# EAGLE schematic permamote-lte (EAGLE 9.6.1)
AUTHOR: NEAL JACKSON; REV: C; TITLE: PERMAMOTE

## Sheet 1 of 5: NRF
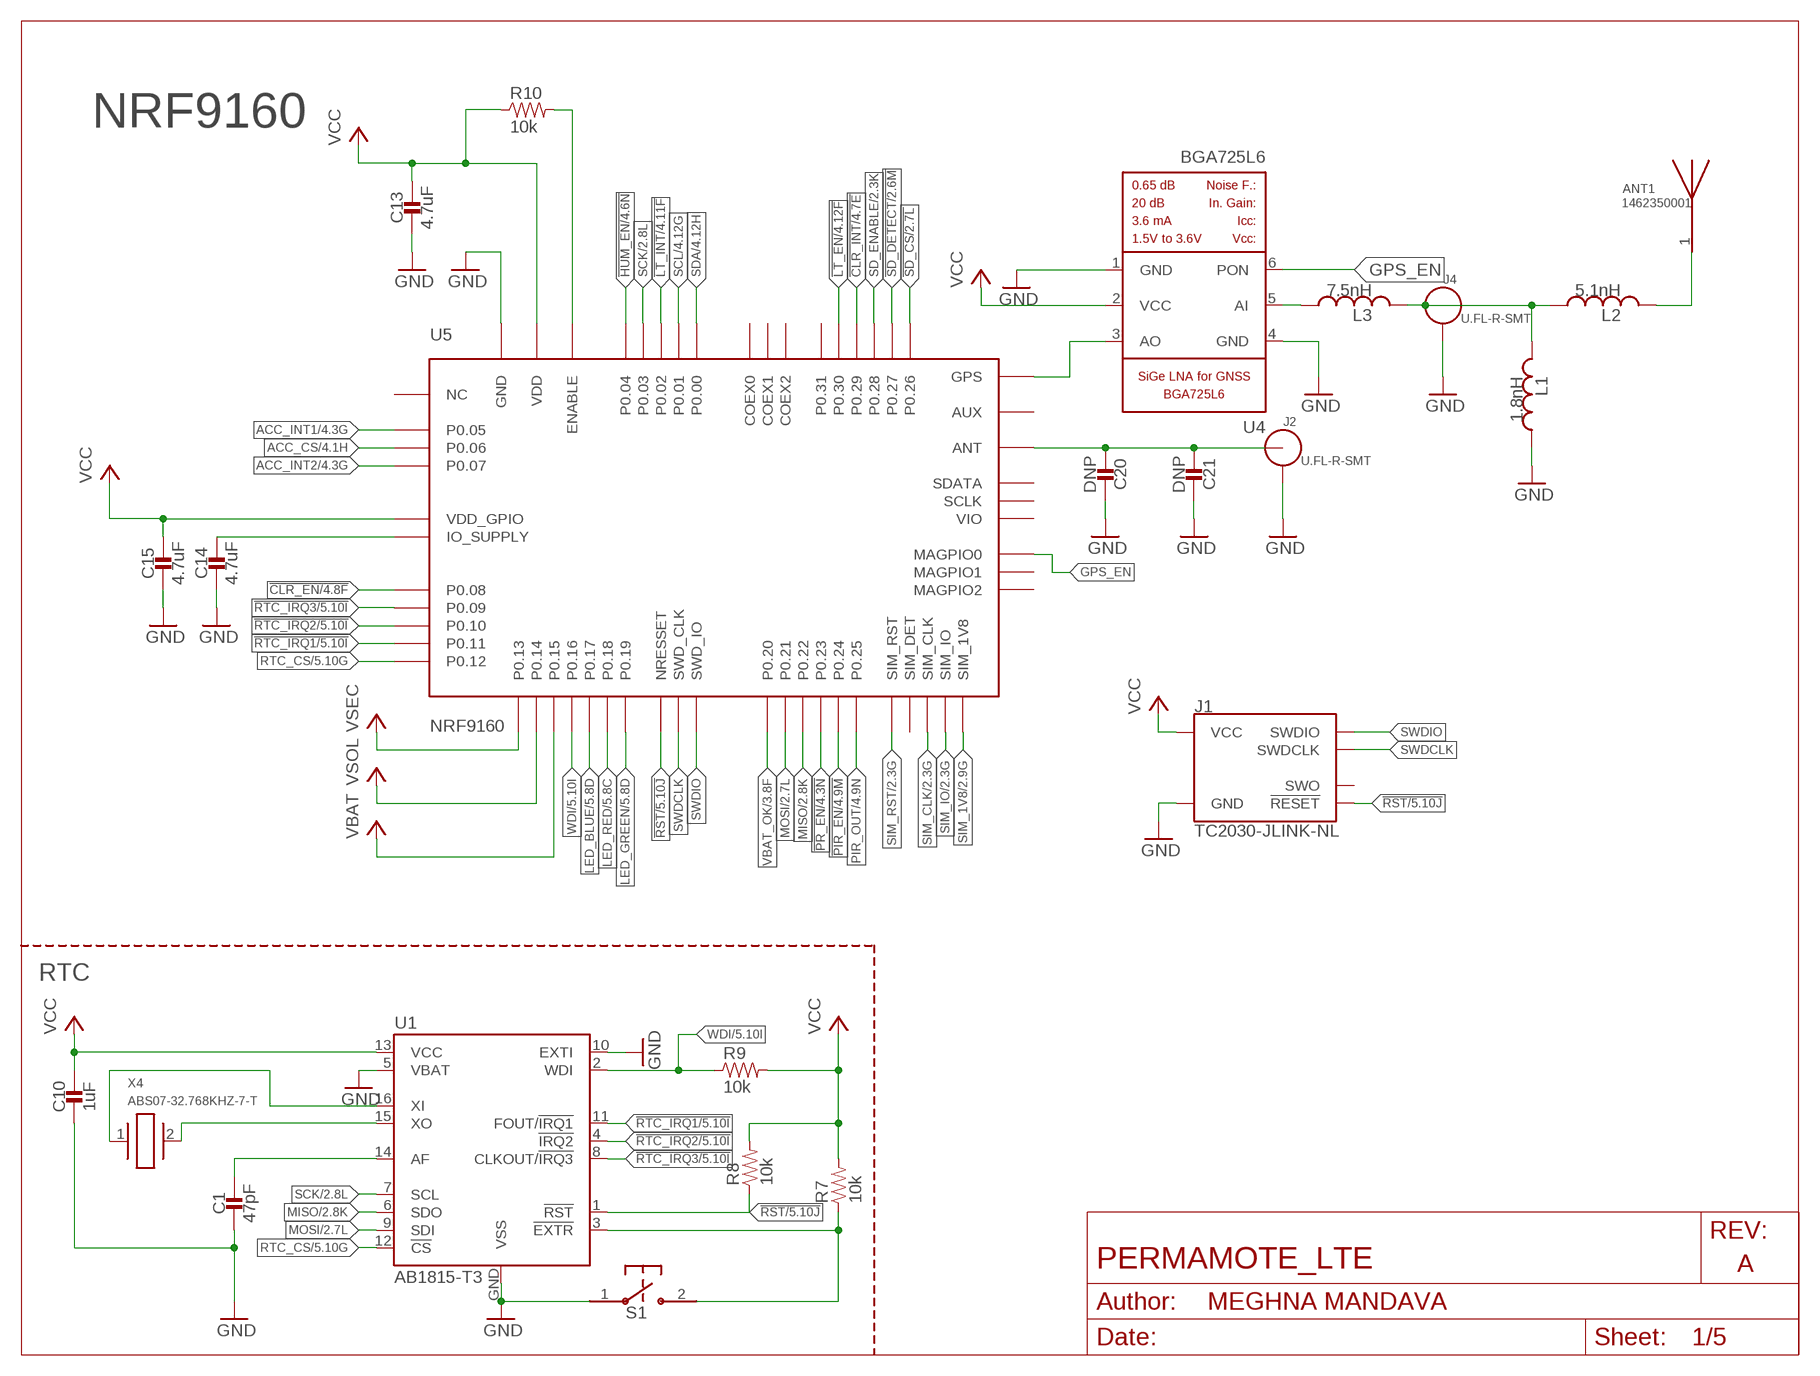
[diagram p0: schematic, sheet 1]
FRAME1 (LETTER_L_BLANK): AUTHOR: MEGHNA MANDAVA; REV: A; TITLE: PERMAMOTE_LTE

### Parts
ANT1  1462350001  [ANT_1462350001]
C1  47pF  CAPACITOR0402_CAP  [0402_CAP]
C10  1uF  CAPACITOR0402_CAP  [0402_CAP]
C13  4.7uF  CAPACITOR0402_CAP  [0402_CAP]
C14  4.7uF  CAPACITOR0402_CAP  [0402_CAP]
C15  4.7uF  CAPACITOR0402_CAP  [0402_CAP]
C20  DNP  CAPACITOR0402_CAP  [0402_CAP]
C21  DNP  CAPACITOR0402_CAP  [0402_CAP]
J1  TC2030-JLINK-NL  [TC2030-IDC-NL]
J2  U.FL-R-SMT  [U.FL_SMT]
J4  U.FL-R-SMT  [U.FL_SMT]
L1  1.8nH  INDUCTOR0402  [0402_CAP]
L2  5.1nH  INDUCTOR0402  [0402_CAP]
L3  7.5nH  INDUCTOR0402  [0402_CAP]
R7  10k  RESISTOR0402_RES  [0402_RES]
R8  10k  RESISTOR0402_RES  [0402_RES]
R9  10k  RESISTOR0402_RES  [0402_RES]
R10  10k  RESISTOR0402_RES  [0402_RES]
S1  B3U-1000P  [B3U-1000P]
U1  AB1815-T3  [QFN-16-3MM]
U4  BGA725L6  [LNA-TSLP-6-2-ORIG]
U5  NRF9160  [NRF9160]
X4  ABS07-32.768KHZ-7-T  [2-SMD]

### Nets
!CLR_EN: U5.P0.08 ; also sheet 4,5
!CLR_INT: U5.P0.29 ; also sheet 4,5
!HUM_EN: U5.P0.04 ; also sheet 4,5
!LT_EN: U5.P0.30 ; also sheet 4,5
!LT_INT: U5.P0.02 ; also sheet 4,5
!PIR_EN: U5.P0.24 ; also sheet 4,5
!PR_EN: U5.P0.23 ; also sheet 4,5
!RST: J1.3(!RESET) R8.1 U1.1(!RST) U5.NRESET(NRESSET) ; also sheet 5
!RTC_EXTR: R7.1 S1.2 U1.3(!EXTR)
!RTC_IRQ1: U1.11(FOUT/!IRQ1) U5.P0.11 ; also sheet 5
!RTC_IRQ2: U1.4(!IRQ2) U5.P0.10 ; also sheet 5
!RTC_IRQ3: U1.8(CLKOUT/!IRQ3) U5.P0.09 ; also sheet 5
!SD_CS: U5.P0.26 ; also sheet 2
!SD_DETECT: U5.P0.27 ; also sheet 2
ACC_CS: U5.P0.06 ; also sheet 4,5
ACC_INT1: U5.P0.05 ; also sheet 4,5
ACC_INT2: U5.P0.07 ; also sheet 4,5
GND: C1.2 C10.2 C13.2 C14.2 C15.2 C20.1 C21.1 J1.5(GND) J2.GND1 J2.GND2 J4.GND1 J4.GND2 L1.1 S1.1 U1.5(VBAT) U1.10(EXTI) U1.GND(VSS) U4.1(GND) U4.4(GND) U5.GND@1(GND) U5.GND@2(GND) U5.GND@3(GND) U5.GND@4(GND) U5.GND@5(GND) U5.GND@6(GND) U5.GND@7(GND) U5.GND@8(GND) U5.GND@9(GND) U5.GND@10(GND) U5.GND@11(GND) U5.GND@12(GND) U5.GND@13(GND) U5.GND@14(GND) U5.GND@15(GND) U5.GND@16(GND) U5.GND@17(GND) U5.GND@18(GND) U5.GND@19(GND) U5.GND@20(GND) U5.GND@21(GND) U5.GND@22(GND) U5.GND@23(GND) U5.GND@24(GND) U5.GND@25(GND) U5.GND@26(GND) U5.GND@27(GND) U5.GND@28(GND) U5.GND@29(GND) U5.GND@30(GND) U5.GND@31(GND) U5.GND@32(GND) U5.GND@33(GND) U5.GND@34(GND) U5.GND@35(GND) U5.GND_SHIELD@1(GND) U5.GND_SHIELD@2(GND) U5.GND_SHIELD@3(GND) U5.GND_SHIELD@4(GND) U5.GND_SHIELD@5(GND) U5.GND_SHIELD@6(GND) U5.GND_SHIELD@7(GND) U5.GND_SHIELD@8(GND) U5.GND_SHIELD@9(GND) U5.GND_SHIELD@10(GND) U5.GND_SHIELD@11(GND) U5.GND_SHIELD@12(GND) U5.GND_SHIELD@13(GND) U5.GND_SHIELD@14(GND) U5.GND_SHIELD@15(GND) U5.GND_SHIELD@16(GND) U5.GND_SHIELD@17(GND) U5.GND_SHIELD@18(GND) U5.GND_SHIELD@19(GND) U5.GND_SHIELD@20(GND) U5.GND_SHIELD@21(GND) U5.GND_SHIELD@22(GND) U5.GND_SHIELD@23(GND) U5.GND_SHIELD@24(GND) U5.GND_SHIELD@25(GND) U5.GND_SHIELD@26(GND) U5.GND_SHIELD@27(GND) U5.GND_SHIELD@28(GND) U5.GND_SHIELD@29(GND) U5.GND_SHIELD@30(GND) U5.GND_SHIELD@31(GND) U5.GND_SHIELD@32(GND) U5.GND_SHIELD@33(GND) U5.GND_SHIELD@34(GND) ; also sheet 2,3,4,5
GPS_EN: U4.6(PON) U5.MAGPIO0
LED_BLUE: U5.P0.17 ; also sheet 5
LED_GREEN: U5.P0.19 ; also sheet 5
LED_RED: U5.P0.18 ; also sheet 5
MISO: U1.6(SDO) U5.P0.22 ; also sheet 2,4,5
MOSI: U1.9(SDI) U5.P0.21 ; also sheet 2,4,5
N$1: U4.3(AO) U5.GPS
N$2: L3.1 U4.5(AI)
N$4: J4.SIG(ANT) L1.2 L2.1 L3.2
N$5: ANT1.1 L2.2
N$8: C20.2 C21.2 J2.SIG(ANT) U5.ANT
N$25: C1.1 U1.14(AF)
N$28: R10.2 U5.ENABLE
N$29: C14.1 U5.IO_SUPPLY
N$40: U1.15(XO) X4.2
N$43: U1.16(XI) X4.1
PIR_OUT: U5.P0.25 ; also sheet 4,5
RTC_CS: U1.12(!CS) U5.P0.12 ; also sheet 5
SCK: U1.7(SCL) U5.P0.03 ; also sheet 2,4,5
SCL: U5.P0.01 ; also sheet 4,5
SD_ENABLE: U5.P0.28 ; also sheet 2
SDA: U5.P0.00 ; also sheet 4,5
SIM_1V8: U5.SIM_1V8 ; also sheet 2
SIM_CLK: U5.SIM_CLK ; also sheet 2
SIM_IO: U5.SIM_IO ; also sheet 2
SIM_RST: U5.SIM_RST ; also sheet 2
SWDCLK: J1.4(SWDCLK) U5.SWDCLK(SWD_CLK)
SWDIO: J1.2(SWDIO) U5.SWDIO(SWD_IO)
VBAT: U5.P0.15 ; also sheet 3
VBAT_OK: U5.P0.20 ; also sheet 3
VCC: C10.1 C13.1 C15.1 J1.1(VCC) R7.2 R8.2 R9.2 R10.1 U1.13(VCC) U4.2(VCC) U5.VDD@1(VDD) U5.VDD@2(VDD) U5.VDD_GPIO ; also sheet 2,3,4,5
VSEC: U5.P0.13 ; also sheet 3
VSOL: U5.P0.14 ; also sheet 3,5
WDI: R9.1 U1.2(WDI) U5.P0.16 ; also sheet 5
Unconnected: J1.6(SWO) U5.AUX U5.COEX0 U5.COEX1 U5.COEX2 U5.MAGPIO1 U5.MAGPIO2 U5.NC1(NC) U5.NC2(NC) U5.NC3(NC) U5.NC4(NC) U5.NC5(NC) U5.NC6(NC) U5.NC7(NC) U5.NC8(NC) U5.NC9(NC) U5.NC10(NC) U5.NC11(NC) U5.NC12(NC) U5.NC13(NC) U5.NC14(NC) U5.NC15(NC) U5.NC16(NC) U5.NC17(NC) U5.NC18(NC) U5.NC19(NC) U5.NC20(NC) U5.NC21(NC) U5.NC22(NC) U5.NC23(NC) U5.NC24(NC) U5.NC25(NC) U5.NC26(NC) U5.NC27(NC) U5.NC28(NC) U5.NC29(NC) U5.NC30(NC) U5.NC31(NC) U5.NC32(NC) U5.NC33(NC) U5.NC34(NC) U5.NC35(NC) U5.P0.31 U5.SCLK U5.SDATA U5.SIM_DET U5.VIO

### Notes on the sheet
- NRF9160
- RTC

## Sheet 2 of 5: SIM and SD
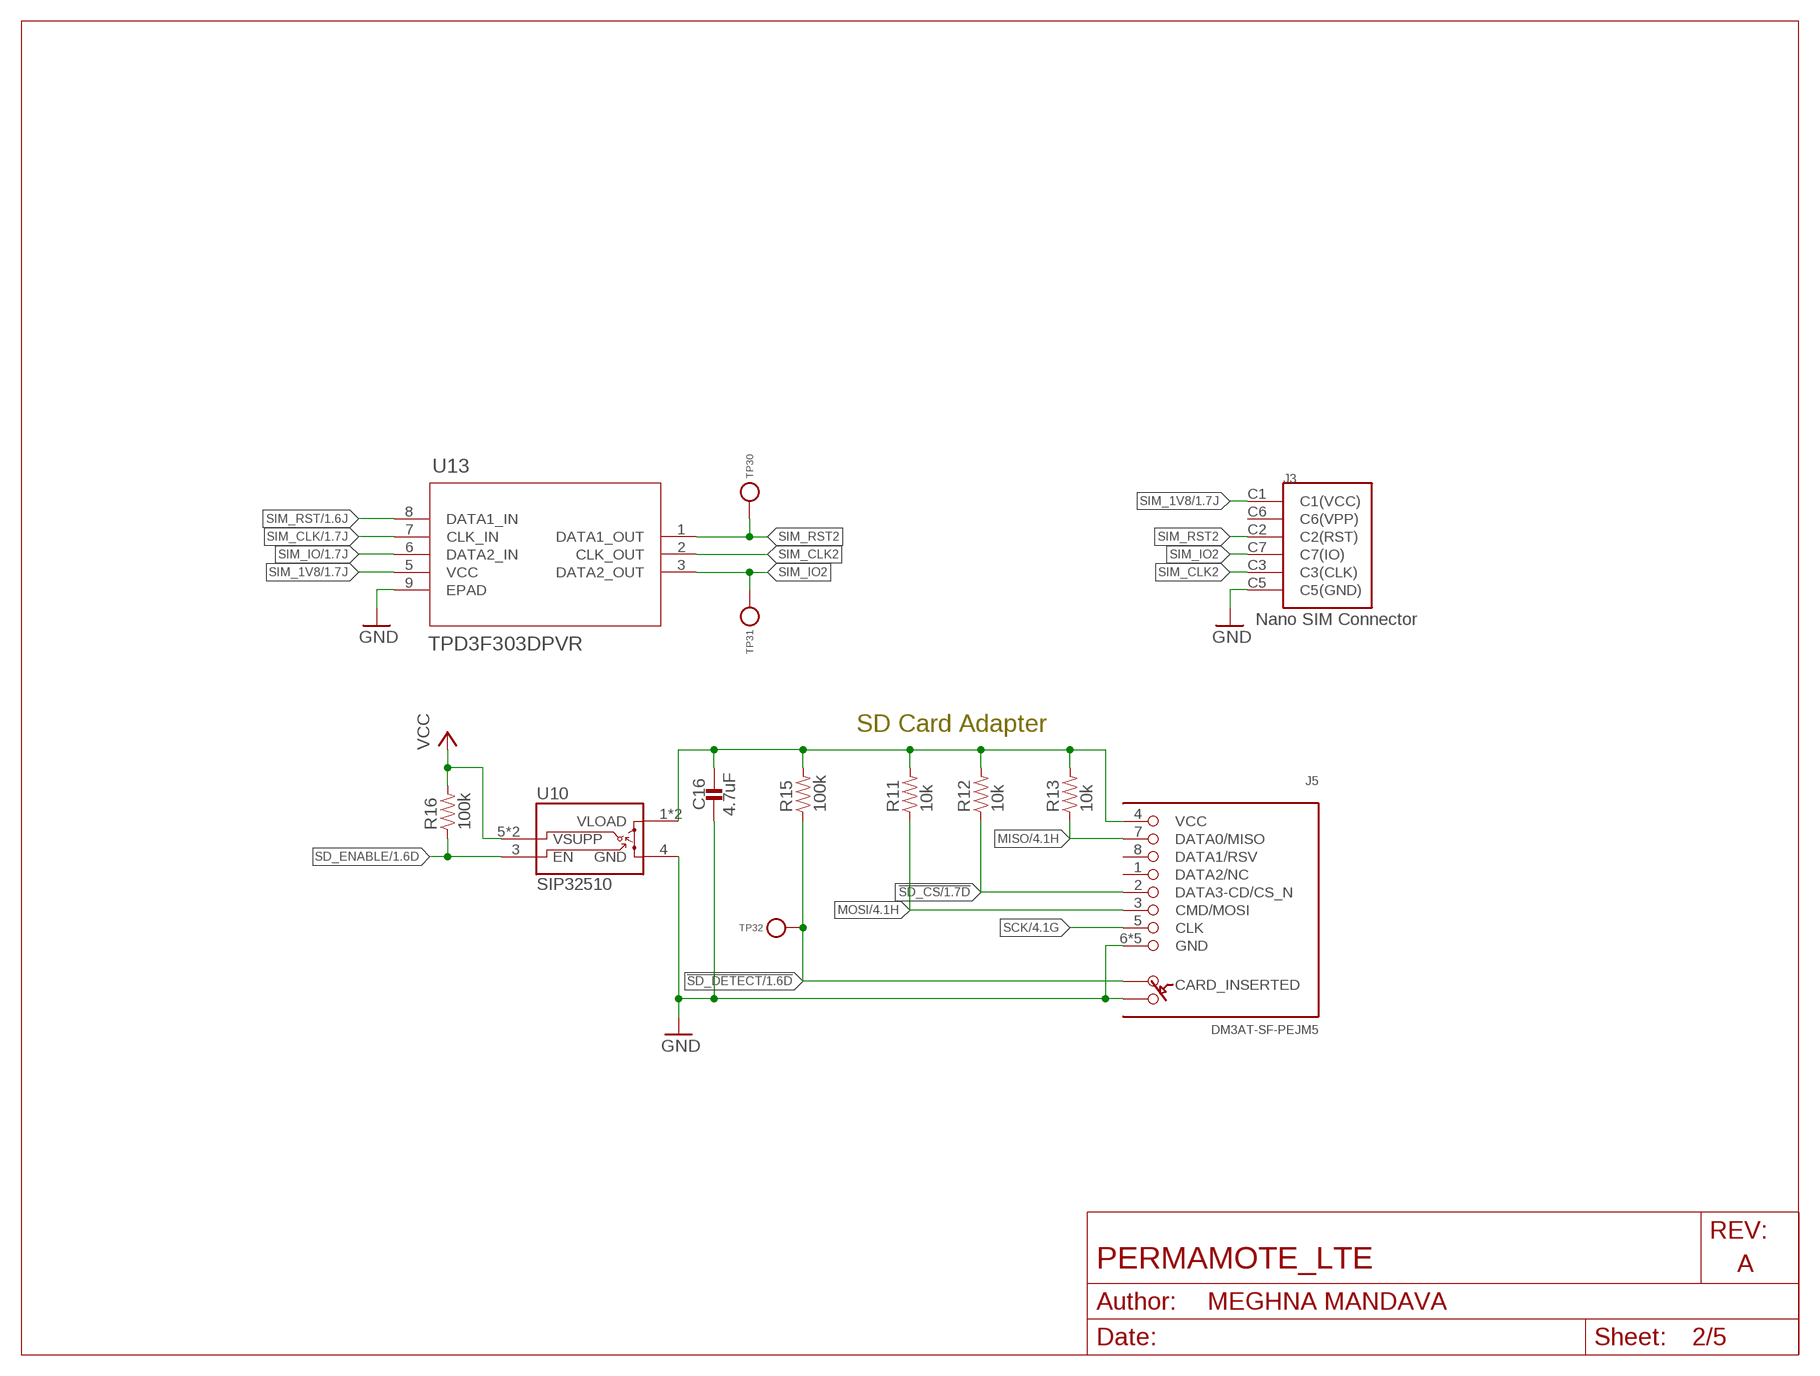
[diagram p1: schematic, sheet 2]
FRAME4 (LETTER_L_BLANK): AUTHOR: MEGHNA MANDAVA; REV: A; TITLE: PERMAMOTE_LTE

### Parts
C16  4.7uF  CAPACITOR0402_CAP  [0402_CAP]
J3  NANO_SIM  [WURTH_NANO_SIM]
J5  DM3AT-SF-PEJM5  [DM3AT-SF-PEJM5]
R11  10k  RESISTOR0402_RES  [0402_RES]
R12  10k  RESISTOR0402_RES  [0402_RES]
R13  10k  RESISTOR0402_RES  [0402_RES]
R15  100k  RESISTOR0402_RES  [0402_RES]
R16  100k  RESISTOR0402_RES  [0402_RES]
TP30  TEST-POINT  [PAD.03X.03]
TP31  TEST-POINT  [PAD.03X.03]
TP32  TEST-POINT  [PAD.03X.03]
U10  SIP32510  [TSOT23-6]
U13  TPD3F303DPVR  [DPV8_1P7X0P4]

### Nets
!SD_CS: J5.2(DATA3-CD/CS_N) R12.1 ; also sheet 1
!SD_DETECT: J5.A R15.1 TP32.P$1(TESTPOINT) ; also sheet 1
GND: C16.2 J3.C5(C5(GND)) J5.6(GND) J5.B J5.MOUNT0(GND) J5.MOUNT1(GND) J5.MOUNT2(GND) J5.MOUNT3(GND) U10.4(GND) U13.9(EPAD) ; also sheet 1,3,4,5
MISO: J5.7(DATA0/MISO) R13.1 ; also sheet 1,4,5
MOSI: J5.3(CMD/MOSI) R11.1 ; also sheet 1,4,5
N$13: C16.1 J5.4(VCC) R11.2 R12.2 R13.2 R15.2 U10.1(VLOAD) U10.2(VLOAD)
SCK: J5.5(CLK) ; also sheet 1,4,5
SD_ENABLE: R16.1 U10.3(EN) ; also sheet 1
SIM_1V8: J3.C1(C1(VCC)) U13.5(VCC) ; also sheet 1
SIM_CLK: U13.7(CLK_IN) ; also sheet 1
SIM_CLK2: J3.C3(C3(CLK)) U13.2(CLK_OUT)
SIM_IO: U13.6(DATA2_IN) ; also sheet 1
SIM_IO2: J3.C7(C7(IO)) TP31.P$1(TESTPOINT) U13.3(DATA2_OUT)
SIM_RST: U13.8(DATA1_IN) ; also sheet 1
SIM_RST2: J3.C2(C2(RST)) TP30.P$1(TESTPOINT) U13.1(DATA1_OUT)
VCC: R16.2 U10.5(VSUPP) U10.6(VSUPP) ; also sheet 1,3,4,5
Unconnected: J3.C6(C6(VPP)) J5.1(DATA2/NC) J5.8(DATA1/RSV)

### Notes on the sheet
- SD Card Adapter

## Sheet 3 of 5: Power supply
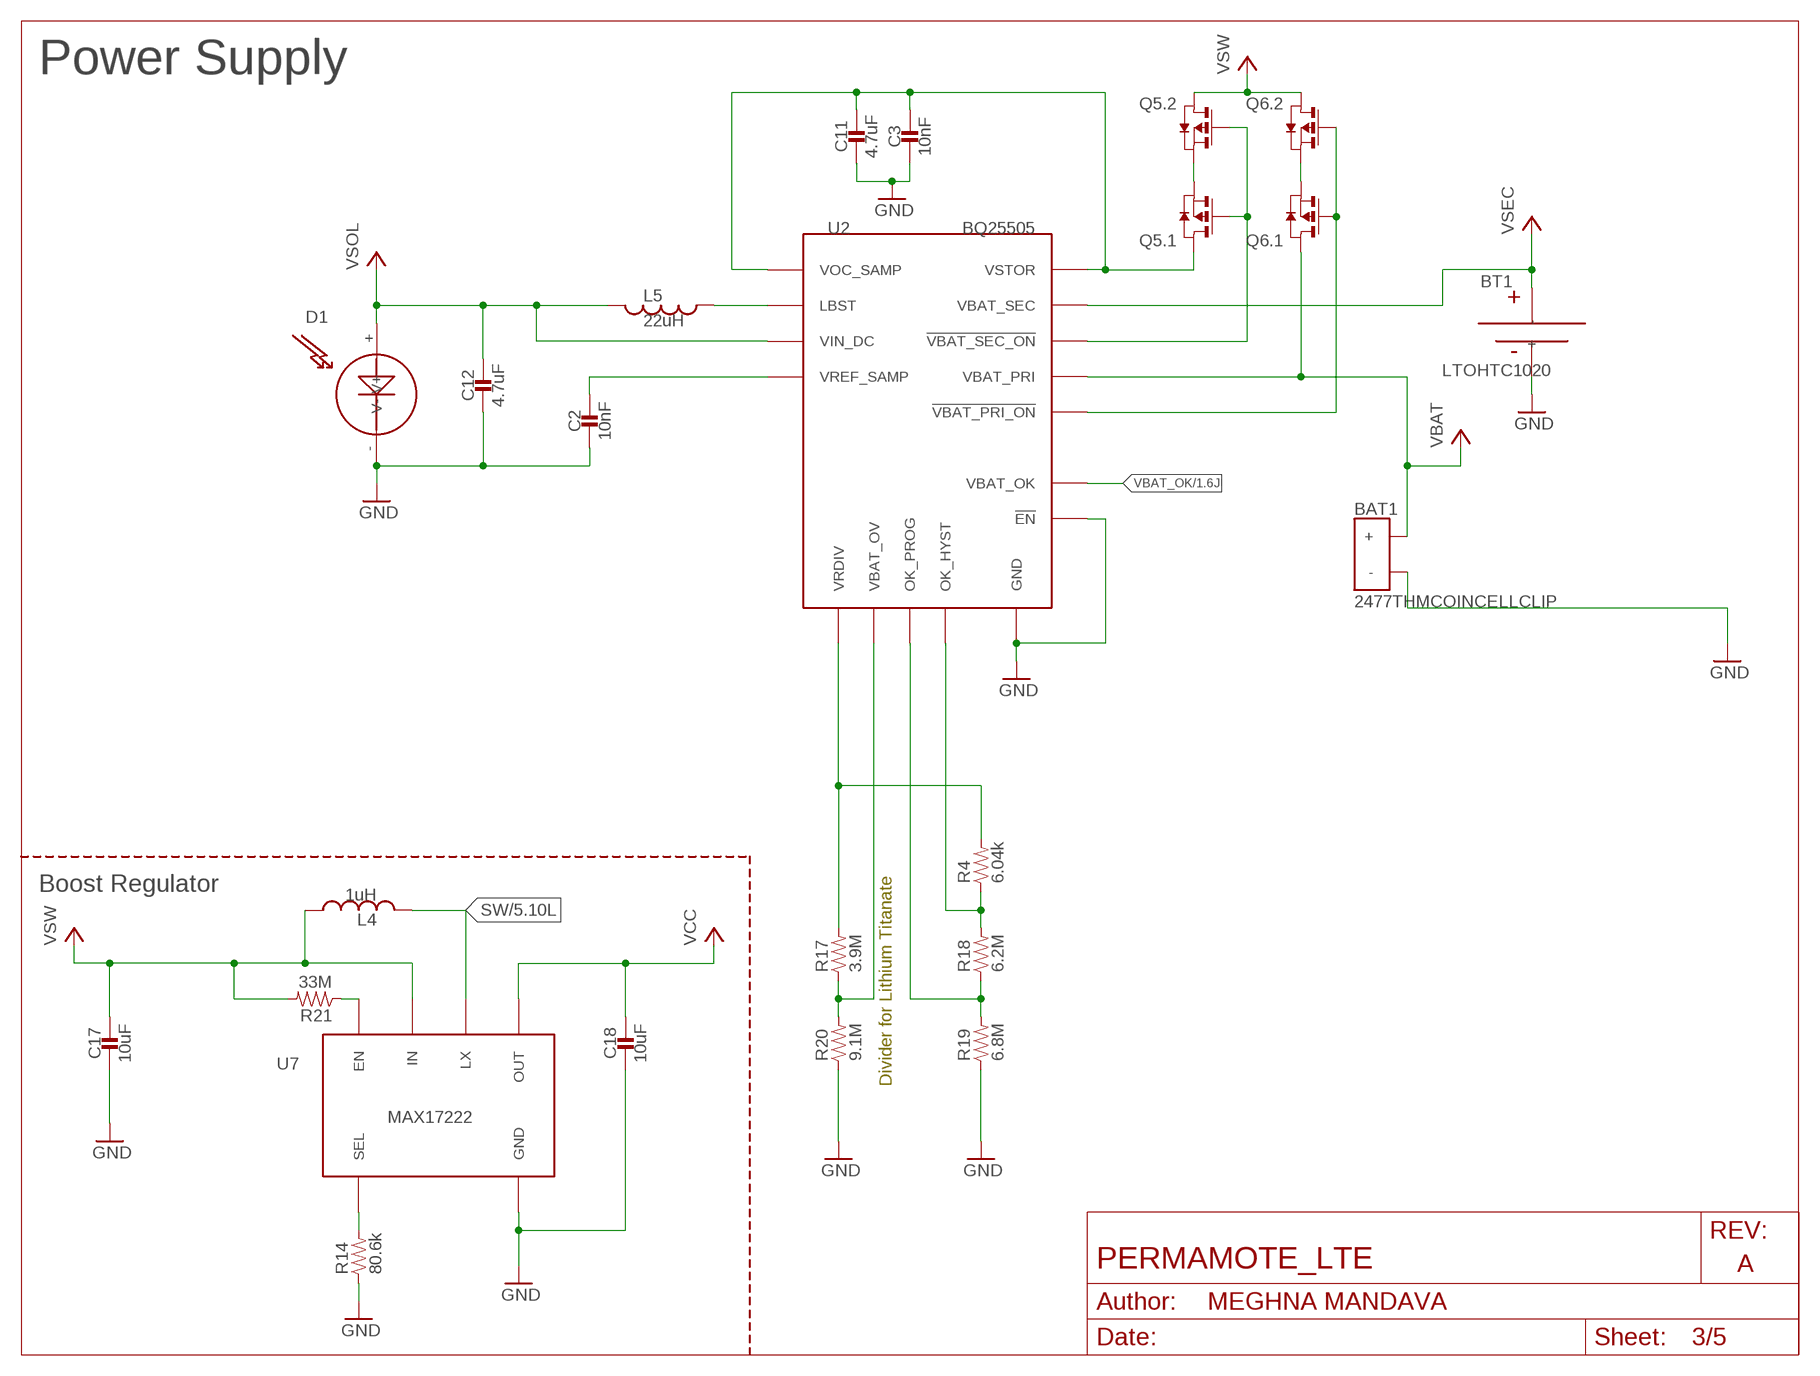
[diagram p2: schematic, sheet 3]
FRAME2 (LETTER_L_BLANK): AUTHOR: MEGHNA MANDAVA; REV: A; TITLE: PERMAMOTE_LTE

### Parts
BAT1  2477THMCOINCELLCLIP  [2477THMCOINCLIP]
BT1  LTOHTC1020  [1020]
C2  10nF  CAPACITOR0402_CAP  [0402_CAP]
C3  10nF  CAPACITOR0402_CAP  [0402_CAP]
C11  4.7uF  CAPACITOR0402_CAP  [0402_CAP]
C12  4.7uF  CAPACITOR0402_CAP  [0402_CAP]
C17  10uF  CAPACITOR0603_CAP  [0603_CAP]
C18  10uF  CAPACITOR0603_CAP  [0603_CAP]
D1  SOLARCELLHOLES  [SOLAR_HOLES]
L4  1uH  INDUCTORIHL  [IHL-1212BZ-11]
L5  22uH  INDUCTOR74437324220  [74437324220]
Q5  PMDXB950UPEL  [XDFN-6]
Q6  PMDXB950UPEL  [XDFN-6]
R4  6.04k  RESISTOR0402_RES  [0402_RES]
R14  80.6k  RESISTOR0603_RES  [0603-RES]
R17  3.9M  RESISTOR0402_RES  [0402_RES]
R18  6.2M  RESISTOR0402_RES  [0402_RES]
R19  6.8M  RESISTOR0402_RES  [0402_RES]
R20  9.1M  RESISTOR0402_RES  [0402_RES]
R21  33M  RESISTOR0603_RES  [0603-RES]
U2  BQ25505  [S-PVQFN-N20-RGR]
U7  MAX17222  [UDFN-6-MAXIM]

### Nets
!VBAT_PRI_ON: Q6.2(.1:G) Q6.5(.2:G) U2.10(!VBAT_PRI_ON)
!VBAT_SEC_ON: Q5.2(.1:G) Q5.5(.2:G) U2.9(!VBAT_SEC_ON)
GND: BAT1.GND(-) BT1.- C2.2 C3.2 C11.2 C12.2 C17.2 C18.2 D1.-(V-) R14.1 R19.1 R20.1 U2.1(GND) U2.5(!EN) U2.6(GND) U2.15(GND) U2.16(GND) U2.17(GND) U2.PAD(GND) U7.3(GND) ; also sheet 1,2,4,5
LBST: L5.P$1 U2.20(LBST)
N$12: R14.2 U7.4(SEL)
N$14: R21.1 U7.6(EN)
N$18: R17.1 R20.2 U2.7(VBAT_OV)
N$32: R4.2 R17.2 U2.8(VRDIV)
N$45: Q5.1(.1:S) Q5.4(.2:S)
N$53: Q6.1(.1:S) Q6.4(.2:S)
N$57: R18.1 R19.2 U2.12(OK_PROG)
N$58: R4.1 R18.2 U2.11(OK_HYST)
SW: L4.P$2 U7.2(LX) ; also sheet 5
VBAT: BAT1.1(+) BAT1.2(+) Q6.6(.1:D) U2.14(VBAT_PRI) ; also sheet 1
VBAT_OK: U2.13(VBAT_OK) ; also sheet 1
VCC: C18.1 U7.1(OUT) ; also sheet 1,2,4,5
VOC_SAMP_VSTOR: C3.1 C11.1 Q5.6(.1:D) U2.3(VOC_SAMP) U2.19(VSTOR)
VREF_SAMP: C2.1 U2.4(VREF_SAMP)
VSEC: BT1.+ U2.18(VBAT_SEC) ; also sheet 1
VSOL: C12.1 D1.+(V+) L5.P$2 U2.2(VIN_DC) ; also sheet 1,5
VSW: C17.1 L4.P$1 Q5.3(.2:D) Q6.3(.2:D) R21.2 U7.5(IN)

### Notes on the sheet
- Power Supply
- Boost Regulator
- Divider for Lithium Titanate

## Sheet 4 of 5: Sensors
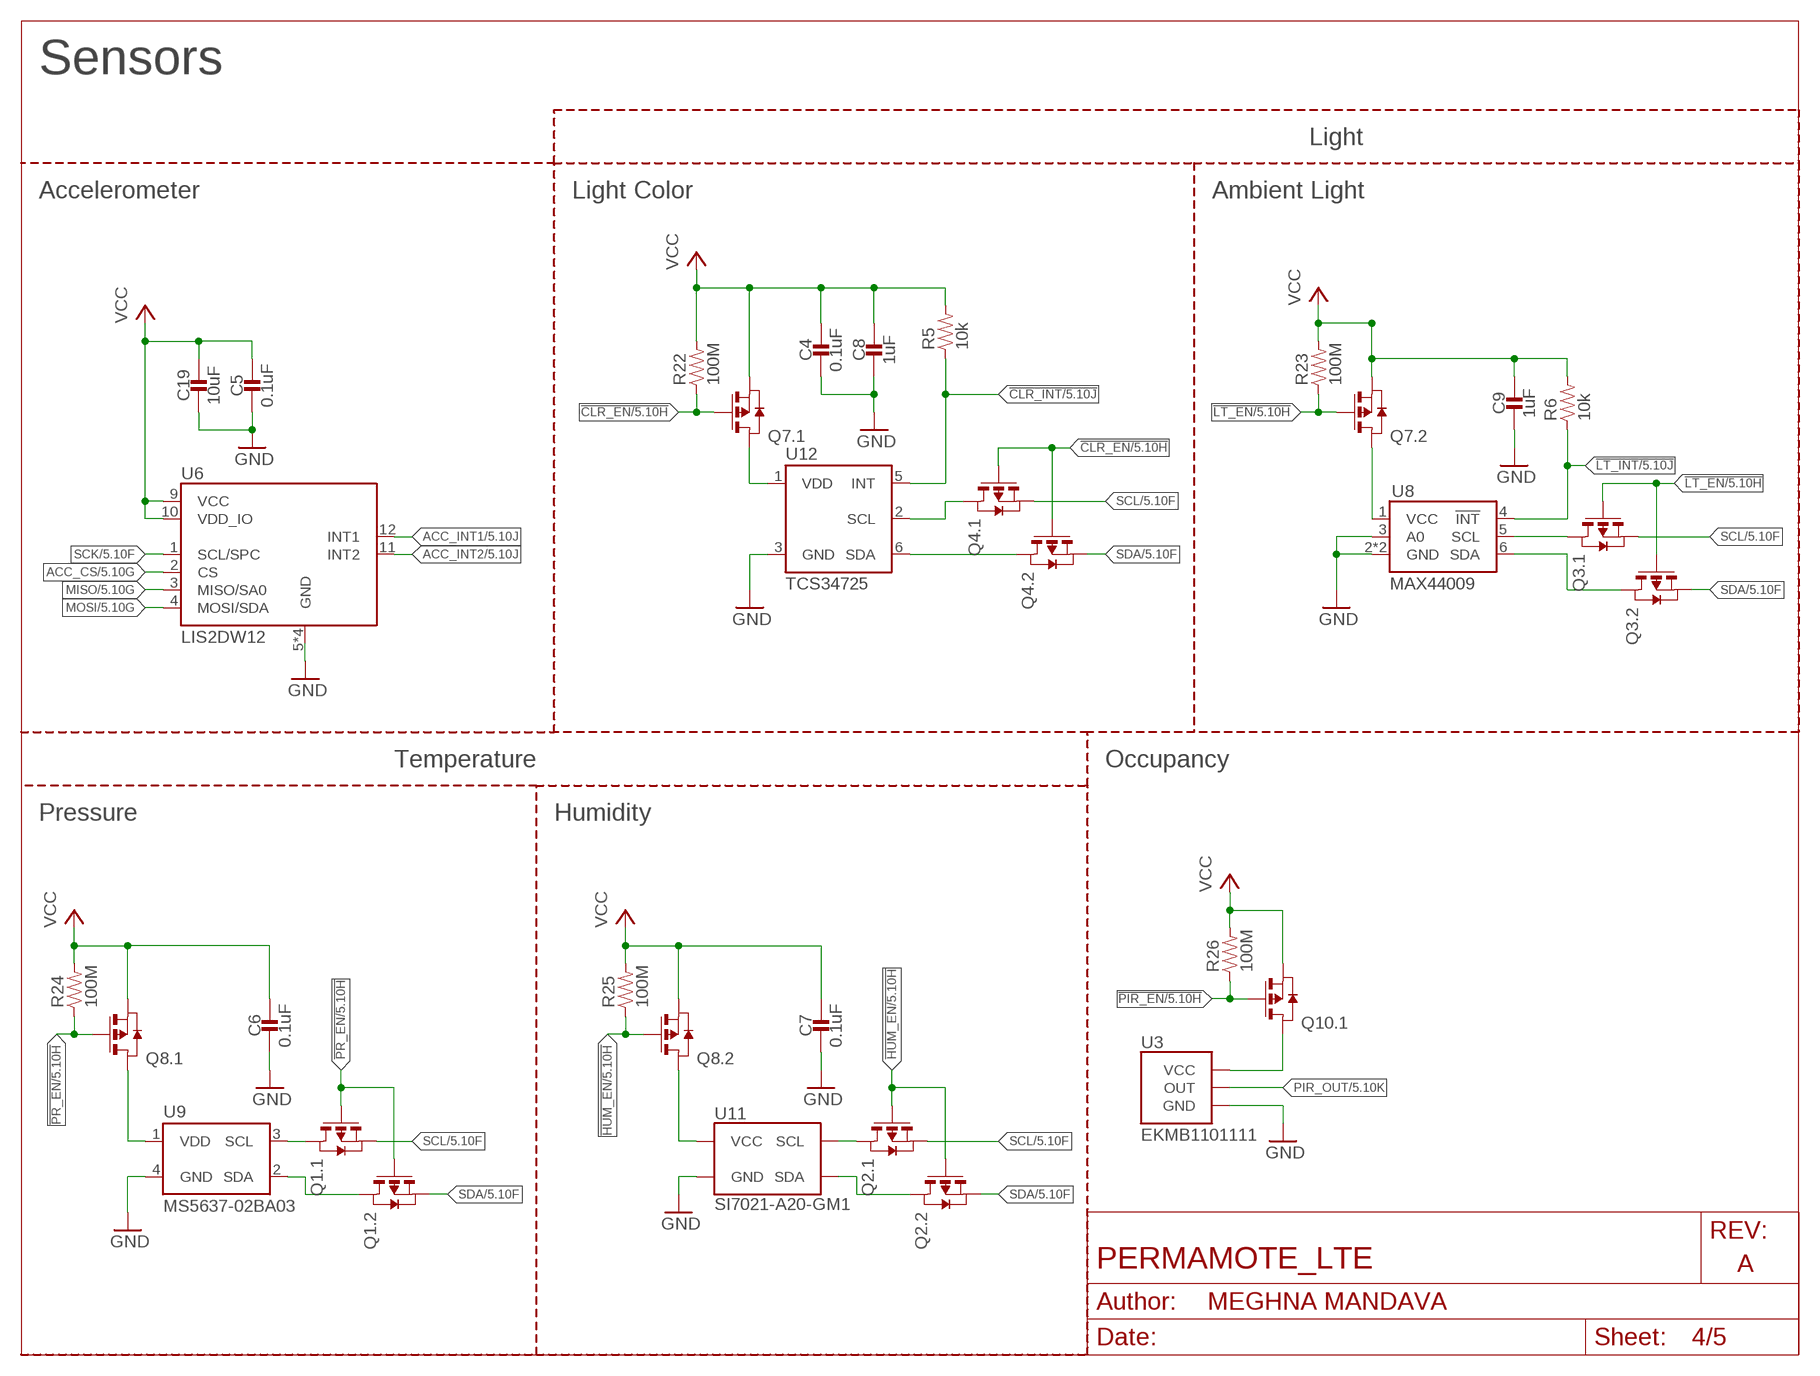
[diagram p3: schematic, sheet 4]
FRAME3 (LETTER_L_BLANK): AUTHOR: MEGHNA MANDAVA; REV: A; TITLE: PERMAMOTE_LTE

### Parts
C4  0.1uF  CAPACITOR0402_CAP  [0402_CAP]
C5  0.1uF  CAPACITOR0402_CAP  [0402_CAP]
C6  0.1uF  CAPACITOR0402_CAP  [0402_CAP]
C7  0.1uF  CAPACITOR0402_CAP  [0402_CAP]
C8  1uF  CAPACITOR0402_CAP  [0402_CAP]
C9  1uF  CAPACITOR0402_CAP  [0402_CAP]
C19  10uF  CAPACITOR0603_CAP  [0603_CAP]
Q1  PMDXB950UPEL  [XDFN-6]
Q2  PMDXB950UPEL  [XDFN-6]
Q3  PMDXB950UPEL  [XDFN-6]
Q4  PMDXB950UPEL  [XDFN-6]
Q7  PMDXB950UPEL  [XDFN-6]
Q8  PMDXB950UPEL  [XDFN-6]
Q10  PMDXB950UPEL  [XDFN-6]
R5  10k  RESISTOR0402_RES  [0402_RES]
R6  10k  RESISTOR0402_RES  [0402_RES]
R22  100M  RESISTOR0402_RES  [0402_RES]
R23  100M  RESISTOR0402_RES  [0402_RES]
R24  100M  RESISTOR0402_RES  [0402_RES]
R25  100M  RESISTOR0402_RES  [0402_RES]
R26  100M  RESISTOR0402_RES  [0402_RES]
U3  EKMB1101111  [AMN2]
U6  LIS2DW12  [LGA-12]
U8  MAX44009  [UDFN-6-EXPOSED]
U9  MS5637-02BA03  [4-SMD]
U11  SI7021-A20-GM1  [DFN-6/3MM]
U12  TCS34725  [FN-6]

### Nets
!CLR_EN: Q4.2(.1:G) Q4.5(.2:G) Q7.2(.1:G) R22.1 ; also sheet 1,5
!CLR_INT: R5.1 U12.5(INT) ; also sheet 1,5
!HUM_EN: Q2.2(.1:G) Q2.5(.2:G) Q8.5(.2:G) R25.1 ; also sheet 1,5
!LT_EN: Q3.2(.1:G) Q3.5(.2:G) Q7.5(.2:G) R23.1 ; also sheet 1,5
!LT_INT: R6.1 U8.4(!INT) ; also sheet 1,5
!PIR_EN: Q10.2(.1:G) R26.1 ; also sheet 1,5
!PR_EN: Q1.2(.1:G) Q1.5(.2:G) Q8.2(.1:G) R24.1 ; also sheet 1,5
ACC_CS: U6.2(CS) ; also sheet 1,5
ACC_INT1: U6.12(INT1) ; also sheet 1,5
ACC_INT2: U6.11(INT2) ; also sheet 1,5
GND: C4.2 C5.2 C6.2 C7.2 C8.2 C9.2 C19.2 U3.GND U6.5(GND) U6.6(GND) U6.7(GND) U6.8(GND) U8.2(GND) U8.3(A0) U8.EP(GND) U9.4(GND) U11.2(GND) U12.3(GND) ; also sheet 1,2,3,5
MISO: U6.3(MISO/SA0) ; also sheet 1,2,5
MOSI: U6.4(MOSI/SDA) ; also sheet 1,2,5
N$20: Q7.3(.2:D) U8.1(VCC)
N$21: Q8.6(.1:D) U9.1(VDD)
N$22: Q8.3(.2:D) U11.5(VCC)
N$23: Q10.6(.1:D) U3.VCC
N$31: Q7.6(.1:D) U12.1(VDD)
N$34: Q1.6(.1:D) U9.3(SCL)
N$41: Q1.3(.2:D) U9.2(SDA)
N$48: Q2.3(.2:D) U11.1(SDA)
N$50: Q2.6(.1:D) U11.6(SCL)
N$51: Q3.3(.2:D) U8.6(SDA)
N$52: Q3.6(.1:D) U8.5(SCL)
N$54: Q4.3(.2:D) U12.6(SDA)
N$55: Q4.6(.1:D) U12.2(SCL)
PIR_OUT: U3.OUT ; also sheet 1,5
SCK: U6.1(SCL/SPC) ; also sheet 1,2,5
SCL: Q1.1(.1:S) Q2.1(.1:S) Q3.1(.1:S) Q4.1(.1:S) ; also sheet 1,5
SDA: Q1.4(.2:S) Q2.4(.2:S) Q3.4(.2:S) Q4.4(.2:S) ; also sheet 1,5
VCC: C4.1 C5.1 C6.1 C7.1 C8.1 C9.1 C19.1 Q7.1(.1:S) Q7.4(.2:S) Q8.1(.1:S) Q8.4(.2:S) Q10.1(.1:S) R5.2 R6.2 R22.2 R23.2 R24.2 R25.2 R26.2 U6.9(VCC) U6.10(VDD_IO) ; also sheet 1,2,3,5
Unconnected: Q10.3(.2:D) Q10.4(.2:S) Q10.5(.2:G)

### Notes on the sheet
- Sensors
- Light
- Accelerometer | Light Color | Ambient Light
- Temperature | Occupancy
- Pressure | Humidity

## Sheet 5 of 5: Debugging
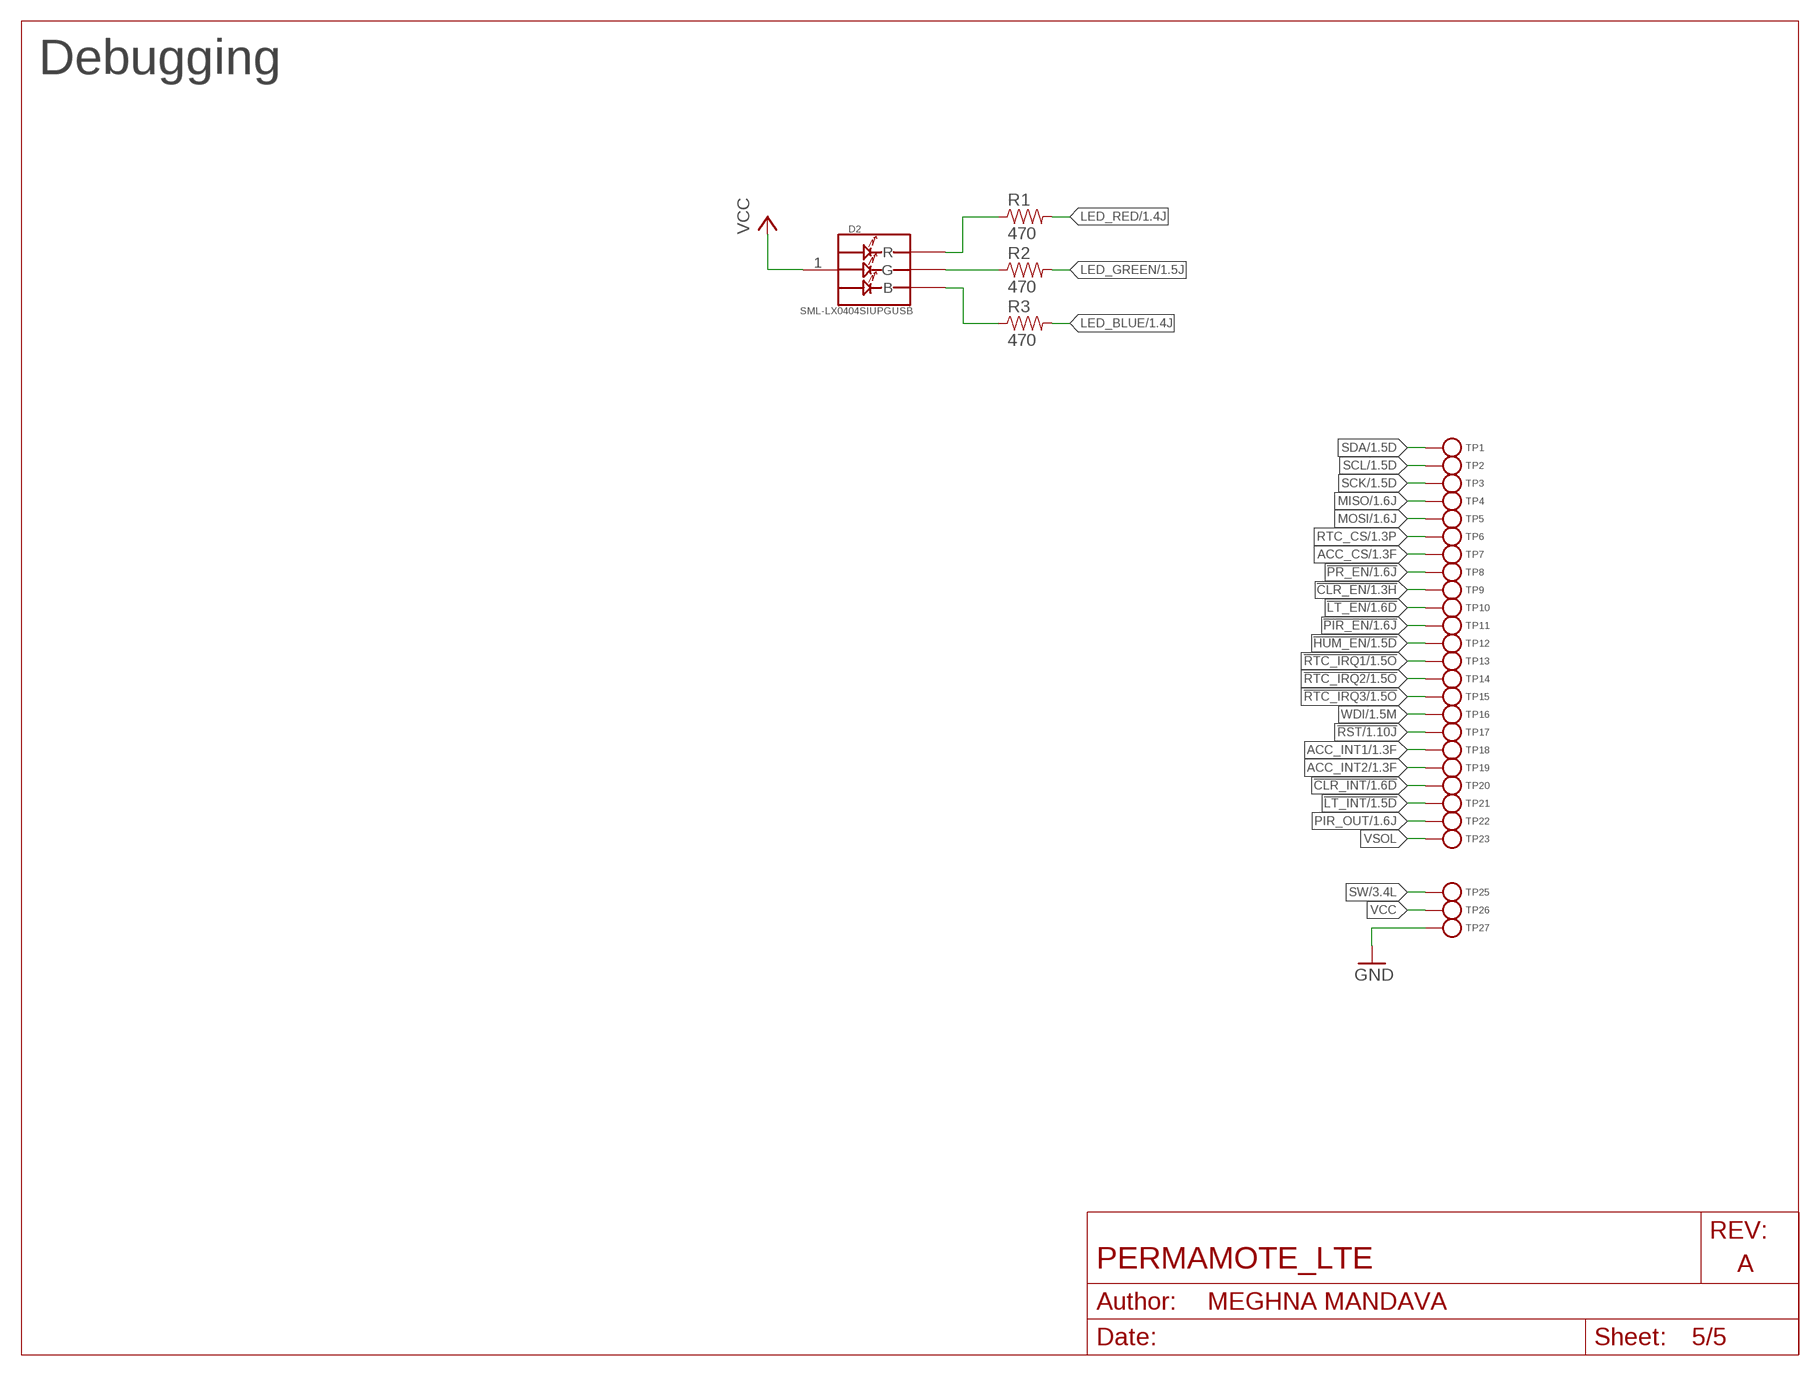
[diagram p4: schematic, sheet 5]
FRAME5 (LETTER_L_BLANK): AUTHOR: MEGHNA MANDAVA; REV: A; TITLE: PERMAMOTE_LTE

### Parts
D2  SML-LX0404SIUPGUSB  [1MM_SQ_4PAD]
R1  470  RESISTOR0402_RES  [0402_RES]
R2  470  RESISTOR0402_RES  [0402_RES]
R3  470  RESISTOR0402_RES  [0402_RES]
TP1  TEST-POINT  [PAD.03X.03]
TP2  TEST-POINT  [PAD.03X.03]
TP3  TEST-POINT  [PAD.03X.03]
TP4  TEST-POINT  [PAD.03X.03]
TP5  TEST-POINT  [PAD.03X.03]
TP6  TEST-POINT  [PAD.03X.03]
TP7  TEST-POINT  [PAD.03X.03]
TP8  TEST-POINT  [PAD.03X.03]
TP9  TEST-POINT  [PAD.03X.03]
TP10  TEST-POINT  [PAD.03X.03]
TP11  TEST-POINT  [PAD.03X.03]
TP12  TEST-POINT  [PAD.03X.03]
TP13  TEST-POINT  [PAD.03X.03]
TP14  TEST-POINT  [PAD.03X.03]
TP15  TEST-POINT  [PAD.03X.03]
TP16  TEST-POINT  [PAD.03X.03]
TP17  TEST-POINT  [PAD.03X.03]
TP18  TEST-POINT  [PAD.03X.03]
TP19  TEST-POINT  [PAD.03X.03]
TP20  TEST-POINT  [PAD.03X.03]
TP21  TEST-POINT  [PAD.03X.03]
TP22  TEST-POINT  [PAD.03X.03]
TP23  TEST-POINT  [PAD.03X.03]
TP25  TEST-POINT  [PAD.03X.03]
TP26  TEST-POINT  [PAD.03X.03]
TP27  TEST-POINT  [PAD.03X.03]

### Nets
!CLR_EN: TP9.P$1(TESTPOINT) ; also sheet 1,4
!CLR_INT: TP20.P$1(TESTPOINT) ; also sheet 1,4
!HUM_EN: TP12.P$1(TESTPOINT) ; also sheet 1,4
!LT_EN: TP10.P$1(TESTPOINT) ; also sheet 1,4
!LT_INT: TP21.P$1(TESTPOINT) ; also sheet 1,4
!PIR_EN: TP11.P$1(TESTPOINT) ; also sheet 1,4
!PR_EN: TP8.P$1(TESTPOINT) ; also sheet 1,4
!RST: TP17.P$1(TESTPOINT) ; also sheet 1
!RTC_IRQ1: TP13.P$1(TESTPOINT) ; also sheet 1
!RTC_IRQ2: TP14.P$1(TESTPOINT) ; also sheet 1
!RTC_IRQ3: TP15.P$1(TESTPOINT) ; also sheet 1
ACC_CS: TP7.P$1(TESTPOINT) ; also sheet 1,4
ACC_INT1: TP18.P$1(TESTPOINT) ; also sheet 1,4
ACC_INT2: TP19.P$1(TESTPOINT) ; also sheet 1,4
GND: TP27.P$1(TESTPOINT) ; also sheet 1,2,3,4
LED_BLUE: R3.2 ; also sheet 1
LED_GREEN: R2.2 ; also sheet 1
LED_RED: R1.2 ; also sheet 1
MISO: TP4.P$1(TESTPOINT) ; also sheet 1,2,4
MOSI: TP5.P$1(TESTPOINT) ; also sheet 1,2,4
N$15: D2.2(R) R1.1
N$17: D2.4(G) R2.1
N$19: D2.3(B) R3.1
PIR_OUT: TP22.P$1(TESTPOINT) ; also sheet 1,4
RTC_CS: TP6.P$1(TESTPOINT) ; also sheet 1
SCK: TP3.P$1(TESTPOINT) ; also sheet 1,2,4
SCL: TP2.P$1(TESTPOINT) ; also sheet 1,4
SDA: TP1.P$1(TESTPOINT) ; also sheet 1,4
SW: TP25.P$1(TESTPOINT) ; also sheet 3
VCC: D2.1(VDD) TP26.P$1(TESTPOINT) ; also sheet 1,2,3,4
VSOL: TP23.P$1(TESTPOINT) ; also sheet 1,3
WDI: TP16.P$1(TESTPOINT) ; also sheet 1

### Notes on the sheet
- Debugging

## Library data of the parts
ANT1 = chips:1462350001: Antenna GPS 1.4dBi Gain 1578MHz SMD T/R; DESCRIPTION: Antenna GPS 1.4dBi Gain 1578MHz SMD T/R; DIGI-KEY_PART_NUMBER: WM15009CT-ND; DIGI-KEY_PURCHASE_URL: https://www.digikey.com/product-detail/en/molex/1462350001/WM15009CT-ND/6159255?utm_source=snapeda&utm_medium=aggregator&utm_campaign=symbol; DIGIKEY: WM15009CT-ND; MF: Molex; MP: 1462350001; MPN: 1462350001; PACKAGE: None
BAT1 = batteries:2477THMCOINCELLCLIP: Battery clip for 2477 Coin Cell; DIGIKEY: 36-3039-ND; MANUFACTURER: Keystone; MPN: 3039
BT1 = batteries:LTOHTC
C1 = passives:CAPACITOR: SMD Capacitor; DIGIKEY: 490-5942-1-ND; MPN: GRM1555C1H470JA01D
C2 C3 = passives:CAPACITOR: SMD Capacitor; DIGIKEY: 490-4516-1-ND; MPN: GRM155R71H103KA88D
C4-C7 = passives:CAPACITOR: SMD Capacitor; DIGIKEY: 490-6328-1-ND; MPN: GRM155R71C104KA88J
C8-C10 = passives:CAPACITOR: SMD Capacitor; DIGIKEY: 490-7195-1-ND; MPN: GRM155R70G105KA12D
C11-C15 = passives:CAPACITOR: SMD Capacitor; DIGIKEY: 445-5947-1-ND; MPN: C1005X5R0J475K050BC
C16 = passives:CAPACITOR: SMD Capacitor; DESCRIPTION: CAP CER 4.7UF 10V X5R 0402; DIGIKEY: 1276-1480-1-ND; MANUFACTURER: Samsung Electro-Mechanics; MPN: CL05A475KP5NRNC
C17-C19 = passives:CAPACITOR: SMD Capacitor; DIGIKEY: 490-3896-1-ND; MPN: GRM188R60J106ME47D
C20 C21 = passives:CAPACITOR: SMD Capacitor
D1 = permamote:SOLARCELL: Generic solar cell; DIGIKEY: 869-1001-ND; MPN: AM-1454CA
D2 = leds:SML-LX0404SIUPGUSB: 1mm^2 RGB LED; DIGIKEY: 67-2125-1-ND; MANUFACTURER: Lumex Opto; MPN: SML-LX0404SIUPGUSB
J1 = connector:TC2030-JLINK
J2 J4 = connector:U.FL-R-SMT: U.FL-R-SMT Antenna Connector; DIGIKEY: H122041-ND; MANUFACTURER: Hirose; MPN: U.FL-R-SMT-1(01)
J3 = signpost:NANO_SIM: WURTH Nano SIM Connector; DIGIKEY: 732-5954-1-ND; MANUFACTURER: Wurth; MPN: 693043020611
J5 = connector:DM3AT-SF-PEJM5: CONN MICRO SD R/A PUSH-PUSH SMD; DESCRIPTION: CONN MICRO SD CARD PUSH-PUSH R/A; DIGIKEY: HR1964CT-ND; MANUFACTURER: Hirose Electric Co Ltd; MPN: DM3AT-SF-PEJM5
L1 = passives:INDUCTOR: A very specific inductor; DIGIKEY: 490-2613-1-ND; MPN: LQG15HS1N8S02D
L2 = passives:INDUCTOR: A very specific inductor; DIGIKEY: 490-6564-1-ND; MPN: LQG15HN5N1S02D
L3 = passives:INDUCTOR: A very specific inductor; DIGIKEY: 490-6565-1-ND; MPN: LQG15HN7N5J02D
L4 = passives:INDUCTOR: A very specific inductor; DIGIKEY: 541-1319-1-ND; MANUFACTURER: Vishay Dale; MPN: IHLP1212BZER1R0M11
L5 = passives:INDUCTOR: A very specific inductor; DIGIKEY: 732-3340-1-ND; MPN: 74437324220
Q1-Q8 Q10 = fets:PMDXB950UPEL: 20 V 500mA, dual P-channel Trench MOSFET; DIGIKEY: 1727-2601-1-ND; MANUFACTURER: NEXPERIA; MPN: PMDXB950UPELZ
R1-R3 = passives:RESISTOR: Resistor; DIGIKEY: 311-470JRCT-ND; MPN: RC0402JR-07470RL
R4 = passives:RESISTOR: Resistor; DIGIKEY: YAG2293CT-ND; MPN: RC0402FR-076K04L
R5-R10 = passives:RESISTOR: Resistor; DIGIKEY: 311-10KJRCT-ND; MPN: RC0402JR-0710KL
R11-R13 = passives:RESISTOR: Resistor; DESCRIPTION: RES SMD 10K OHM 1% 1/16W 0402; DIGIKEY: 1276-3431-1-ND; MANUFACTURER: Samsung Electro-Mechanics; MPN: RC1005F103CS
R14 = passives:RESISTOR: Resistor; DIGIKEY: 311-80.6KHRCT-ND; MPN: RC0603FR-0780K6L
R15 R16 = passives:RESISTOR: Resistor; DESCRIPTION: RES SMD 100K OHM 1% 1/5W 0402; DIGIKEY: 541-100KYCT-ND; MANUFACTURER: Vishay Dale; MPN: CRCW0402100KFKEDHP
R17 = passives:RESISTOR: Resistor; DIGIKEY: YAG3301CT-ND; MPN: RC0402JR-073M9L
R18 = passives:RESISTOR: Resistor; DIGIKEY: YAG3309CT-ND; MPN: RC0402JR-076M2L
R19 = passives:RESISTOR: Resistor; DIGIKEY: YAG3310CT-ND; MPN: RC0402JR-076M8L
R20 = passives:RESISTOR: Resistor; DIGIKEY: YAG3322CT-ND; MPN: RC0402JR-079M1L
R21 = passives:RESISTOR: Resistor; DIGIKEY: HMC0603JT33M0CT-ND; MPN: HMC0603JT33M0
R22-R26 = passives:RESISTOR: Resistor; DIGIKEY: 541-100MAHCT-ND; MPN: HMC0402JT100M
S1 = switches:B3U: Switch; DIGIKEY: SW1020CT-ND; MANUFACTURER: Omron; MPN: B3U-1000P
TP1-TP23 TP25-TP27 TP30-TP32 = headers:TEST-POINT
U1 = chips:AB1815-T3: Ultra-low current RTC. 55nA quiescent @ 3V. 1.5-3.6V input.; DIGIKEY: 535-11936-1-ND; MANUFACTURER: Abracon; MPN: AB1815-T3
U2 = chips:BQ25505: EH front end for switching between primary and secondary cells; DIGIKEY: 296-37078-1-ND; MANUFACTURER: TI; MPN: BQ25505RGRR
U3 = chips:EKMB: Passive infrared human detection sensor with built-in amp.; DIGIKEY: 255-3065-ND; MANUFACTURER: PANASONIC; MPN: EKMB1101111
U4 = chips:BGA725L6; DIGIKEY: BGA725L6E6327FTSA1CT-ND; MANUFACTURER: Infineon Technologies; MPN: BGA725L6E6327FTSA1
U5 = chips:NRF9160; DIGIKEY: 1490-1076-1-ND; MANUFACTURER: Nordic Semiconductor; MPN: NRF9160-SICA-R7
U6 = chips:LIS2DW12: ultra low power 3 axis accelerometer; DIGIKEY: 497-17718-6-ND; MANUFACTURER: STMicroelectronics; MOUSER: 511-LIS2DW12TR; MPN: LIS2DW12TR
U7 = chips:MAX17222: Very high efficiency, very low power boost converter suitable for EH applications; DIGIKEY: MAX17222ELT+TCT-ND; MANUFACTURER: MAXIM INTEGRATED; MPN: MAX17222ELT+T
U8 = chips:MAX44009: low power ambient light sensor; DIGIKEY: MAX44009EDT+TCT-ND; MANUFACTURER: MAXIM; MPN: MAX44009EDT+T
U9 = chips:MS5637-02BA03: low power pressure sensor; DIGIKEY: 223-1199-1-ND; MANUFACTURER: TE CONNECTIVITY; MPN: MS563702BA03-50
U10 = chips:SIP32510: Load switch, slew rate controlled. By Vishay; DESCRIPTION: IC LOAD SWITCH SOT23-6; DIGIKEY: SIP32510DT-T1-GE3CT-ND; MANUFACTURER: Vishay; MPN: SIP32510DT-T1-GE3
U11 = chips:SI7021: IC TEMP SENSOR RH 2% DFN; DIGIKEY: 336-3141-ND; MOUSER: 634-SI7021-A20-GM1; MPN: SI7021-A20-GM1
U12 = chips:TCS34725: Color Light-to-Digital Converter with IR Filter; DIGIKEY: TCS34725FNCT-ND; MPN: TCS34725FN
U13 = chips:TPD3F303DPVR; DIGIKEY: 296-28299-1-ND; MANUFACTURER_PART_NUMBER: TPD3F303DPVR; MPN: TPD3F303DPVR; VENDOR: Texas Instruments
X4 = crystals:ABS07-32.768KHZ: 32.768kHz Crystal; DIGIKEY: 535-9543-1-ND; MANUFACTURER: ABRACON; MPN: ABS07-32.768KHZ-7-T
